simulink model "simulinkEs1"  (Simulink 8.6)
settings: Solver=ode1  StartTime=0.0  StopTime=15000  FixedStep=1e-2  RelTol=1e-3

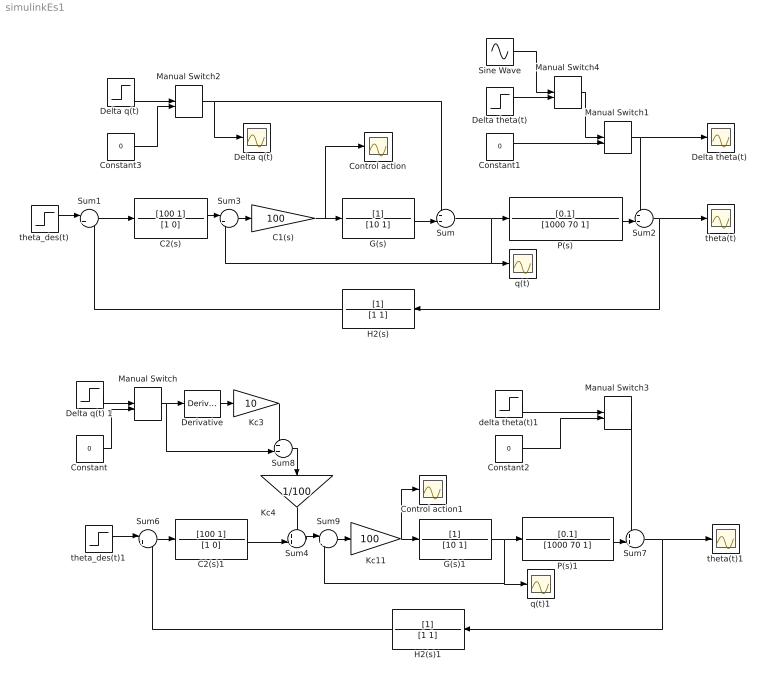
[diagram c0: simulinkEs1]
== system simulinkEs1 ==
  C1(s) : Gain  Gain=100
  C2(s) : TransferFcn  Numerator=[100 1]  Denominator=[1 0]
  C2(s)1 : TransferFcn  Numerator=[100 1]  Denominator=[1 0]
  Constant{,1..3} (4 alike) : Constant  Value=0
  Control action : Scope
  Control action1 : Scope
  "Delta q(t) " : Step  Time=1000  After=-100  SampleTime=0
  "Delta q(t)  " : Scope
  Delta q(t) 1 : Step  Time=1000  After=-100  SampleTime=0
  Delta theta(t) : Step  Time=400  After=5  SampleTime=0
  "Delta theta(t) " : Scope
  Derivative : Derivative
  G(s) : TransferFcn  Denominator=[10 1]
  G(s)1 : TransferFcn  Denominator=[10 1]
  H2(s) : TransferFcn  Denominator=[1 1]
  H2(s)1 : TransferFcn  Denominator=[1 1]
  Kc11 : Gain  Gain=100
  Kc3 : Gain  Gain=10
  Kc4 : Gain  Gain=1/100
  Manual Switch{,1..3} (4 alike) : ManualSwitch
  Manual Switch4 : ManualSwitch  CurrentSetting=0
  P(s) : TransferFcn  Numerator=[0.1]  Denominator=[1000 70 1]
  P(s)1 : TransferFcn  Numerator=[0.1]  Denominator=[1000 70 1]
  Sine Wave : Sin  Amplitude=5  Frequency=1e-3  SampleTime=0
  Sum{,2,4,7..8} (5 alike) : Sum  Inputs=++|
  Sum{1,3,6,9} (4 alike) : Sum  Inputs=|+-
  delta theta(t)1 : Step  Time=400  After=5  SampleTime=0
  q(t) : Scope
  q(t)1 : Scope
  theta(t) : Scope
  theta(t)1 : Scope
  theta_des(t) : Step  Time=0  After=30  SampleTime=0
  theta_des(t)1 : Step  Time=0  After=30  SampleTime=0
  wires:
  G(s)/1 -> Sum/2
  Sum/1 -> q(t)/1, Sum3/2, P(s)/1
  P(s)/1 -> Sum2/2
  Sum2/1 -> theta(t)/1, H2(s)/1
  H2(s)/1 -> Sum1/2
  Sum1/1 -> C2(s)/1
  C1(s)/1 -> Control action/1, G(s)/1
  C2(s)/1 -> Sum3/1
  Sum3/1 -> C1(s)/1
  theta_des(t)/1 -> Sum1/1
  Delta q(t) 1/1 -> Manual Switch/1
  Manual Switch2/1 -> "Delta q(t)  "/1, Sum/1
  C2(s)1/1 -> Sum4/2
  Manual Switch/1 -> Sum8/2, Derivative/1
  Derivative/1 -> Kc3/1
  Kc3/1 -> Sum8/1
  Sum8/1 -> Kc4/1
  Constant/1 -> Manual Switch/2
  G(s)1/1 -> q(t)1/1, Sum9/2, P(s)1/1
  P(s)1/1 -> Sum7/2
  Sum7/1 -> H2(s)1/1, theta(t)1/1
  H2(s)1/1 -> Sum6/2
  Sum6/1 -> C2(s)1/1
  Kc11/1 -> Control action1/1, G(s)1/1
  Sum9/1 -> Kc11/1
  theta_des(t)1/1 -> Sum6/1
  delta theta(t)1/1 -> Manual Switch3/1
  Manual Switch3/1 -> Sum7/1
  Constant2/1 -> Manual Switch3/2
  Sum4/1 -> Sum9/1
  Kc4/1 -> Sum4/1
  "Delta q(t) "/1 -> Manual Switch2/1
  Constant3/1 -> Manual Switch2/2
  Manual Switch1/1 -> "Delta theta(t) "/1, Sum2/1
  Sine Wave/1 -> Manual Switch4/1
  Delta theta(t)/1 -> Manual Switch4/2
  Manual Switch4/1 -> Manual Switch1/1
  Constant1/1 -> Manual Switch1/2
